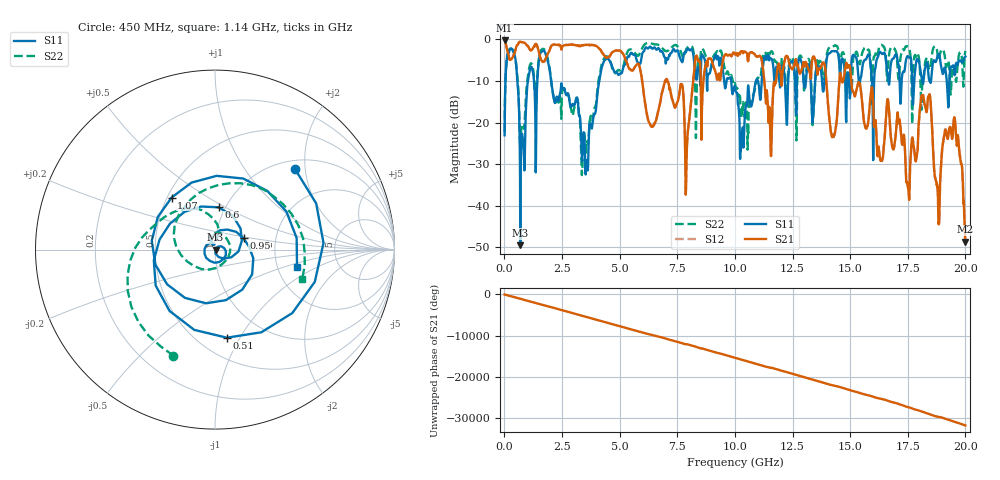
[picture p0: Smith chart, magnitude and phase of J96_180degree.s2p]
!Keysight Technologies,N5222A,MY51421036,A.10.65.16
!Date: Friday, March 31, 2023 14:24:06
!Correction: S11(Full 2 Port(1,2))
!S21(Full 2 Port(1,2))
!S12(Full 2 Port(1,2))
!S22(Full 2 Port(1,2))
!S2P File: Measurements: S11, S21, S12, S22:
# Hz S  dB  R 50
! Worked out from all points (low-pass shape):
!   2000 points, 10 MHz to 20 GHz, reference 50 ohm
!   highest |S21| = -0.24 dB at 10 MHz (marker M1); lowest = -48.7 dB at 20 GHz (marker M2)
!   |S21| within 3 dB of the highest: 436.2 MHz to 1.505 GHz (1.069 GHz wide, 110 % of centre); 1.906 GHz to 4.248 GHz (2.341 GHz wide, 76.1 % of centre)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
!   lowest |S11| = -49.5 dB at 690 MHz (marker M3), VSWR 1.01, Z = 50.3 + j0.0175 ohm
!   |S11| at or under -10 dB: 559.3 MHz to 1.02 GHz (460.3 MHz wide, 58.3 % of centre); 2.026 GHz to 4.114 GHz (2.088 GHz wide, 68 % of centre); 9.84 GHz to 10.92 GHz (1.082 GHz wide, 10.4 % of centre)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
!   |S22| runs from -32.6 to -0.8 dB; largest |S21 - S12| = 0.011
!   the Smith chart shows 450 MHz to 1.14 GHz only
!   S11 on the Smith chart (normalised r, x): 450 MHz: 1.18, +1.76; 510 MHz: 0.68, -0.88; 600 MHz: 0.93, +0.46; 950 MHz: 1.36, +0.18; 1.07 GHz: 0.53, +0.36; 1.14 GHz: 2.57, -0.64
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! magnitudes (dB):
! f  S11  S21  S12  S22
! 10 MHz  -23.1  -0.2  -0.3  -22.2
! 450 MHz  -4.0  -3.1  -3.1  -4.0
! 510 MHz  -6.1  -1.9  -1.9  -5.9
! 600 MHz  -12.5  -1.0  -1.0  -11.5
! 690 MHz  -49.5  -0.6  -0.6  -26.1
! 950 MHz  -15.3  -1.3  -1.3  -12.3
! 1.07 GHz  -8.5  -2.1  -2.1  -7.1
! 1.14 GHz  -6.6  -2.6  -2.6  -5.8
! 3.35 GHz  -26.8  -1.4  -1.4  -31.4
! 6.68 GHz  -2.1  -17.0  -17.0  -1.3
! 7.92 GHz  -2.5  -25.8  -25.7  -2.1
! 10.01 GHz  -11.4  -3.6  -3.6  -10.6
! 11.53 GHz  -4.4  -21.2  -21.3  -3.2
! 13.34 GHz  -17.2  -5.5  -5.5  -16.5
! 14.25 GHz  -2.8  -23.1  -23.0  -1.7
! 14.89 GHz  -8.1  -6.8  -6.8  -10.2
! 16.67 GHz  -10.4  -15.9  -15.8  -4.7
! 17.51 GHz  -4.0  -35.6  -35.6  -1.7
! 18.43 GHz  -9.8  -13.3  -13.3  -7.3
! 18.8 GHz  -3.9  -36.3  -36.4  -3.8
! 19.57 GHz  -6.6  -21.0  -20.8  -9.3
! 20 GHz  -4.1  -48.7  -49.7  -2.8
